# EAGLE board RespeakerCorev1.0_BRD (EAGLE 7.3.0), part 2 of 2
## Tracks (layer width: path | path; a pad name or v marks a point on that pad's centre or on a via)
!PWR_ON  (via drill 0.25 pad 0.51)
  Top 0.152: J6.P$14 J6.14 61.1,28.72 61.4,29.02 61.4,30.67 60.64,31.43 60.64,41.08 57.84,43.88 v57.46,43.88
  Bottom 0.152: v57.46,43.88 57.84,44.26 57.84,49.59 57.43,50.01 Q4.3 56.83,51.52 R4.1 D20.+ 54.65,52.08 Q3.1 54.53,51.09 C27.1
AGND  (via drill 0.25 pad 0.51)
  Top 0.203: U8.8 48.71,21.6 v48.95,21.84 | U8.7 48.9,21.2 v48.95,21.15 | U8.3 46.96,20.42 46.8,20.26 46.29,20.26 v46.16,20.38
  Top 0.406: 44.38,20.87 C68.1 44.41,21.38 v44.38,21.4 44.41,21.42 C69.1 | C29.1 48.93,23.58 48.95,23.56 | 48.95,23.56 48.95,23.58 | 48.95,23.69 48.95,23.58 | 48.95,23.58 R31.1 | 48.95,23.56 48.95,22.65 | C37.1 38.56,27.47 v38.41,27.62 | v45.78,25.21 45.78,24.6 C28.1 | R30.1 C28.1 | C28.1
  Top 0.508: MIC1.2 MIC1.3 | 48.99,21.88 R47.1 50.45,21.88 v50.48,21.91 | 48.99,21.88 v48.95,21.84 | 48.95,22.65 48.95,21.92 48.99,21.88
  Top 0.61: J2.4 39.09,1.63 v40.32,2.86 | J2.3 44.56,2.43 v43.75,3.24 | v38.41,27.62 38.41,28.05 MIC1.3 | MIC1.2 35.83,27.75 C18.1
  Top 1.016: J6.13 J6.P$13
  GND 1.016: J6.P$13 49.89,28.72 49.72,28.89
  Bottom 0.254: U5.28 37.65,38.92 v37.4,38.67
  Bottom 0.406: v45.27,46.42 45.29,46.4 R34.2 47.03,46.4 v47.05,46.42 48.07,45.4 v48.07,45.28 | C24.1 42.22,35.88 v42.35,35.75 | U4.1 v47.81,41.97 | v47.81,41.97 | C15.1 48.07,42.23 v47.81,41.97 | C15.1 v47.3,42.74 46.54,43.5 C14.1 | C15.1 v48.07,43.5 | v48.07,43.5 | C16.1 v48.07,43.5 | v48.07,43.5 | C16.1 v48.07,45.28 | v48.07,45.28 | C14.1 v46.16,44.51 | v46.16,44.51 | C14.1 | v44.64,44.51 C13.1 C14.1 | v44.64,44.51 | C14.1 | v44.64,44.51 v46.16,44.51 | v46.16,44.51 47.94,44.51 C16.1 | C54.2 42.73,40.96 v42.6,41.08 | C38.1 C39.1
  Bottom 0.508: C55.1 v42.6,41.08 | C54.2 v43.49,39.81
  Bottom 0.61: v40.83,33.08 40.8,33.11 C53.1 39.53,32.45 C52.2 38.92,31.46 C39.1 | C38.1 38.54,30.06 38.54,27.75 v38.41,27.62
  other vias: 35.87,38.67 34.35,38.67 34.35,40.2 35.87,40.2 37.4,40.2 37.4,37.15 35.87,37.15 34.35,37.15
  pour GND (isolate 0.254): 39.94,2.6 44.38,2.6 44.38,12.38 51.24,19.24 51.24,43.04 47.22,47.05 40.76,47.05 33.94,40.23 33.94,36.39 44.13,26.19 44.13,16.33 39.94,12.13
AVDD  (via drill 0.25 pad 0.51)
  Top 0.203: U8.1 46.21,21.6 v45.91,21.91
  Top 0.406: v45.91,21.91 C69.2 | v35.62,24.83 35.9,24.83 R58.1
  PWR 0.61: v49.59,43.62 v49.59,41.97 | v49.59,41.97 | 42.29,33.27 42.73,33.72 | 42.73,33.72 49.59,40.58 v49.59,41.97 | v41.46,34.1 41.84,33.72 | 41.84,33.72 42.29,33.27 | 41.84,32.83 35.62,26.61 v35.62,24.83 | 41.84,32.83 42.29,33.27 | 41.84,32.83 41.84,33.72 | 41.84,33.72 42.73,33.72
  Bottom 0.254: U5.32 39.68,36.92
  Bottom 0.406: 40.7,35.9 40.7,35.12 TP4.T | 40.7,35.9 39.68,36.92 | C24.2 40.7,35.9 | v35.62,24.83 41.72,24.83 44.38,22.16 45.65,22.16 v45.91,21.91
  Bottom 0.61: C16.2 v49.59,43.62 C15.2 | C15.2 | U4.2 v49.59,41.97 C15.2 | C15.2 | TP4.T v41.46,34.1
GND  (via drill 0.25 pad 0.51)
  Top 0.152: LC4.1 26.56,65.68 arc-90 26.6,65.72 26.48,65.72 v28.19,66.48 | LC4.2 v27.11,62.8
  Top 0.254: C65.1 27.21,27.77 26.35,28.64 20,28.64 18.98,27.62 18.98,26.23 19.24,25.97 C64.1 18.62,25.82 v18.6,25.84 | v24.63,10.86 24.63,11.3 22.79,13.14 22.49,13.14 | C41.1 22.25,12.92 v22.48,13.14
  Top 0.305: D7.2 27.11,8.32 v26.73,8.7 | D6.2 28.51,8.32 v28.89,8.7 | U7.5 23.69,20.52 v24.19,21.02 | U7.43 22.19,20.29 v22.92,21.02 | U7.15 25.73,21.29 v25.46,21.02 | U7.23 26.69,26 v26.98,26.29 | U7.33 21.69,25.8 21.52,25.97 v21.27,25.97 | U7.35 22.19,24.29 v22.92,23.56 | 30.98,27.05 v30.92,26.99 30.83,26.9 Q1.2 | C67.1 17.9,20.7 v17.84,20.76 | v17.84,20.76 17.84,20.19 17.71,20.07 | v17.84,20.76 17.84,21.4
  Top 0.406: C17.1 33.12,10.69 v33.08,10.73
  Top 0.5: 14.66,61.47 15.03,61.73 arc-20 15.2,61.81 v15.55,61.91
  Top 0.508: C62.1 23.96,16.17 24.77,15.35 | C65.1 27.21,26.52 v26.98,26.29 | C2.1 30.94,27.01 v30.92,26.99 | U6.31 50.76,32.03 | C67.1 18.37,21.12 v18.22,21.27 | C74.2 25.13,15.35 25.71,15.94 v25.97,15.94 | C45.1 25.31,56.3 v25.59,56.58
  Top 0.61: C74.2 24.77,15.35
  Top 0.813: v47.56,2.35 45.65,2.35 v45.65,3.75 | v36.51,1.71 38.54,1.71 v38.54,2.86
  Bottom 0.254: U5.20 35.62,42.35 v35.49,42.48 | U5.24 37.62,41.69 v37.65,41.72 | U5.9 33.11,36.92 32.83,36.64 v32.83,35.62
  Bottom 0.305: U2.3 18.22,14.29 U2.9 | U2.1 19.22,14.3 18.98,14.54 18.86,14.54 U2.9 | U2.6 18.22,14.79 U2.9 | U1.5 U1.PAD | U1.PAD | U2.9 | Q4.2 57.53,51.21 v57.68,51.36
  Bottom 0.406: C49.2 v41.21,46.16 | C33.1 v39.18,46.55 | 18.86,14.54 19.74,14.54 19.87,14.41 | U2.9 17.2,14.54 | v44.32,59.69 44.51,59.5 44.51,57.85 | C48.1 v30.67,10.48
  Bottom 0.508: C51.1 v42.6,42.1 | R6.1 28.23,14.57 C10.1 28,15.18 v27.24,15.94 | C50.1 v36,45.66 | C56.2 42.68,19.65 C57.2 | C5.1 23.17,7.43 v23.3,7.3 | J7.6 43.44,17.03 v43.49,17.08 | R56.1 37.5,17.74 v37.91,17.34
  Bottom 0.61: 27.62,10.73 27.49,10.86 U1.PAD 23.68,10.86 | J7.G1 48.04,14.52
  other vias: 33.84,47.43 46.92,45.4 45.27,45.4 24.95,34.99 28.38,37.66 24.89,46.99 29.71,58.42 29.97,59.05 31.49,62.61 41.4,59.56 46.48,59.69 48.64,55.5 51.94,52.45 51.81,51.05 51.94,49.02 51.81,47.5 60.07,47.5 52.13,32.51 25.71,10.86 20.13,31.69 6.66,36.26 8.31,28.77 9.01,43.31 18.47,14.54 16.44,16.19 13.65,16.32 13.65,15.3 17.14,14.54 19.81,14.41 15.62,10.22 21.08,13.14 26.54,10.92 32.06,14.8 31.43,5.52 24.7,5.4 58.86,17.08 64.58,17.59 58.23,22.8 58.23,24.07 5.52,17.59 6.28,16.19 8.7,21.4 50.16,16 20.76,8.32 44.57,49.4 63.69,16.19 26.86,1.33 23.3,35.75 26.73,48.45 29.14,10.48 49.65,57.98 60.45,54.04 52.83,15.94 57.91,10.86 19.81,5.78 14.73,8.32 12.19,10.86 7.68,20.38 24.25,43.88 27.94,49.47 52.83,18.48 23.68,4.38 25.08,49.47 24.06,37.66 43.24,48.2 46.67,48.2 26.6,15.94 30.73,19.81 31.43,21.78 24.19,22.29 25.46,22.29 22.92,22.29 25.46,23.56 24.19,23.56 47.75,62.61 43.43,62.48 43.94,63.25 46.99,63.25 17.84,19.62 18.92,9.21 20.25,25.84 57.21,45.15 54.03,54.04 8.38,40.7 6.98,40.07 13.33,45.15 54.61,7.05 29.9,8.95 23.81,10.6 23.3,48.32 49.59,61.66 55.88,57.34 54.61,57.21 62.73,50.23 38.79,55.31 45.97,55.94 6.98,25.46 8.25,27.37 9.01,44.64 11.49,20.13 11.49,24.19 54.03,10.22 18.98,56.83 19.49,55.69 21.01,55.31 22.28,55.31 23.55,55.31 23.55,52.77 22.28,52.77 21.01,52.77 19.74,53.4 18.35,54.17 10.54,49.72 63.43,37.02 64.07,32.07 63.75,31.05 21.65,9.59 21.78,10.99 15.43,16.13 25.78,60.58 24.25,60.07 17.01,59.75 18.16,52.9 20.19,52.39 21.01,51.5 22.28,51.5 23.55,51.5 21.9,59.37 29.52,61.79 52.32,13.78 19.11,63.18 11.74,50.36 14.03,50.36 8.31,23.49 4.5,21.59 5.77,23.56 21.65,43.88 62.35,43.24 63.75,29.27 62.67,26.1 62.29,23.56 61.65,19.11 61.02,13.4 21.71,12.64 21.08,12.38 20.19,13.78 42.6,56.96 17.46,55.31 27.62,61.15 16.95,56.58 18.98,58.48 15.93,57.21 18.98,59.75 15.17,57.85 15.17,58.99 25.21,62.17 23.17,61.4 19.74,61.02 23.43,28.57 27.72,26.72 21.27,60.64 29.02,63.56 59.97,51.74 62.63,52.88 57.93,57.96 28.89,12.83 17.33,62.55 29.97,67.12 32,67.88 28.82,65.09 30.6,65.72 32.51,66.36 30.98,64.2 15.87,59.75 17.14,61.15 15.87,61.02 56.22,49.64 55.9,47.17 57.04,47.17 28.44,57.53 64.54,49.9 36.57,62.99 40.38,64.64 41.91,65.79 38.98,65.79 40.13,67.18 7.3,52.9 4.5,48.07 34.1,32.58 30.92,36.13 31.43,14.8 43.49,19.49 30.92,23.81 30.16,23.81 28.38,38.29 49.4,10.99 20.13,32.45 18.41,32.64 29.52,6.54 30.29,6.54 31.05,6.54 29.9,5.91 30.67,5.91 50.8,53.34 49.65,52.45 50.8,51.56 51.05,49.91 51.05,48.26 49.65,47.37 50.8,46.61 49.84,49.4 49.84,51.05 48.64,52.83 49.27,53.72 47.87,53.72 18.16,51.88 18.79,53.4 36,30.42 36,29.91 48.13,16.26 47.87,13.59 49.14,14.99 48,11.43 48.51,10.67 48.51,9.65 48.26,7.75 46.1,6.6 43.68,6.6 42.03,4.95 37.33,9.4 40,6.48 44.45,11.3 43.18,9.65 32.7,42.1 43.11,36.26 43.11,35.62 26.86,36.26 24.95,37.66 34.6,15.18 33.33,13.91 33.84,23.18 33.84,24.7 33.71,26.73 34.35,28.64 34.86,29.15 34.86,31.69 39.43,28.64
  pour Top (isolate 0.254, rank 6): -2.23,-3.62 71.81,-3.62 71.81,70.42 -2.23,70.42
  pour GND (isolate 0.254, rank 5): -2.23,48.96 -2.23,-4.38 -0.58,-4.38 -0.58,-3.62 71.81,-3.62 71.81,70.42 8.57,70.42 -1.49,70.39 -2.22,70.4 -2.22,62.44 -2.23,50.29 -2.23,49.43
  pour Bottom (isolate 0.254, rank 5): -2.23,70.42 -2.23,-5.65 -0.58,-5.65 -0.58,-3.62 71.81,-3.62 71.81,70.42
  pour Top (isolate 0.254, rank 3, no thermals): 22.92,5.52 32.44,5.52 32.44,-1.84 22.92,-1.84
  pour Top (no thermals): 28.51,64.07 27.62,66.48 32.7,68.39 33.59,66.1
  pour Top (no thermals): 27.75,65.85 28.38,64.07 20.44,61.15 20.13,61.91 19.87,61.85 20.51,60.26 29.46,63.56 28.51,66.23 27.75,65.98
  pour Top (isolate 0.254, rank 4, no thermals): 15.17,60.01 14.16,61.79 19.74,63.69 21.01,60.52
GPIO12/UART_TXD0  (via drill 0.25 pad 0.51)
  Top 0.152: 30.03,30.67 30.03,30.57 U6.19 | J6.4 J6.P$4
  Top 0.203: 30.03,30.67 v30.03,31.31
  PWR 0.152: v60.89,29.27 60.89,36.26 58.43,38.72 J6.P$4
  Bottom 0.152: v30.03,31.31 34.86,26.48 42.35,26.48 45.14,23.69 50.61,23.69 52.43,25.51 58.28,25.51 60.89,28.13 v60.89,29.27
  Bottom 0.203: v30.03,31.31 29.4,31.94 TP16.T
GPIO13/UART_RXD0  (via drill 0.25 pad 0.51)
  Top 0.152: U6.20 31.58,30.64 30.92,31.31 v30.79,31.31 | J6.3 J6.P$3
  PWR 0.152: v60.38,29.91 60.38,36.26 58.86,37.78 56.51,37.78 J6.P$3
  Bottom 0.152: v60.38,29.91 60.38,28.13 58.1,25.84 52.26,25.84 50.48,24.07 45.27,24.07 42.48,26.86 34.98,26.86 30.79,31.05 v30.79,31.31 31.43,31.94 TP17.T
GPIO_0/I2S_ADC  (via drill 0.25 pad 0.51)
  Top 0.152: U6.7 18.98,42.23 17.84,41.08 17.84,40.58 16.95,39.69 13.9,39.69 13.39,39.18 13.39,37.72 J5.P$5 J5.5
  Top 0.203: U6.7 v20.38,42.23 | v20.38,42.23
  PWR 0.203: v20.38,42.23 22.12,40.48 v32.57,40.48
  Bottom 0.203: U5.16 32.64,40.42 v32.57,40.48
GPIO_1/I2S_DAC  (via drill 0.25 pad 0.51)
  Top 0.152: U6.8 18.93,40.53 17.12,38.72 J5.4 J5.P$4
  Top 0.203: U6.8 20.33,40.53 v20.38,40.58
  PWR 0.203: v32.57,39.43 21.52,39.43 v20.38,40.58
  Bottom 0.203: U5.14 v32.58,39.42 v32.57,39.43
GPIO_2/I2S_LRCLK  (via drill 0.25 pad 0.51)
  Top 0.152: U6.9 18.88,38.83 16.78,36.72 J5.6 J5.P$6
  Top 0.203: U6.9 20.28,38.83 v20.38,38.93
  PWR 0.203: v20.38,38.93 v20.38,38.92 v32.07,38.92
  Bottom 0.203: v32.07,38.92 U5.13
GPIO_3/I2S_BCLK  (via drill 0.25 pad 0.51)
  Top 0.152: v20.38,37.91 19.6,37.13 U6.10 18.84,37.13 16.43,34.72 J5.8 J5.P$8
  PWR 0.203: v27.5,38.36 20.83,38.36 v20.38,37.91
  Bottom 0.203: R40.2 29.02,39.94 27.5,38.42 v27.5,38.36
GPIO_4/I2C_SCL  (via drill 0.25 pad 0.51)
  Top 0.152: U6.11 19.04,35.43 16.33,32.72 J5.10 J5.P$10
  Top 0.203: U6.11 20.06,35.43 v20.13,35.5
  Bottom 0.203: U5.17 34.12,41.44 33.97,41.59 32.19,41.59 31.56,42.23 R39.1 30.77,42.51 30.41,42.86 27.68,42.86 21.34,36.52 20.39,36.52 20.13,36.26 v20.13,35.5
GPIO_5/I2C_SDA  (via drill 0.25 pad 0.51)
  Top 0.152: U6.12 18.23,33.73 17.84,33.34 17.84,32.07 16.49,30.72 J5.12 J5.P$12
  Top 0.203: U6.12 20.01,33.73 20.76,34.48 v20.76,37.15
  Bottom 0.203: U5.18 34.62,41.45 34.1,41.97 33.59,41.97 33.21,42.35 R38.1 arc90 33.1,43.24 27.24,43.24 21.14,37.15 v20.76,37.15
GPIO_19/PWM_CH1  (via drill 0.25 pad 0.51)
  Top 0.152: U6.34 49.1,37.13 v48.32,37.91
  Bottom 0.152: BUTTON1.1 39.24,60.96 40.32,59.88 40.32,58.4 43.92,54.8 56.57,54.8 57.09,54.29 R33.1 58.28,53.4 TP15.T 59.58,53.45 61.54,51.49 K2.2 61.54,49.81 K2.1 63.25,48.01 59.11,43.88 59.11,40.7 58.1,39.69 54.03,39.69 52.26,37.91 v48.32,37.91
GPIO_40  (via drill 0.25 pad 0.51)
  Top 0.152: U6.57 26.48,53.78 27.62,52.64 v27.62,51.75
  Bottom 0.152: D21.- 52.38,47.69 48.32,51.75 v27.62,51.75
GPIO_41
  Top 0.152: U6.2 18.85,50.73 17.46,49.34 16.67,48.55 R48.1
GPIO_42  (via drill 0.25 pad 0.51)
  Top 0.152: U6.58 24.78,54.31 24.82,54.35 24.82,54.42 v25.46,55.05
  Bottom 0.152: 53.27,52.3 D20.- 53.23,52.81 51.75,54.29 43.75,54.29 40.38,57.66 R11.1 39.29,58.91 TP6.T 37.17,58.96 35.17,60.96 BUTTON1.2 34.92,60.96 29.02,55.05 v25.46,55.05
GPIO_45/UART_TXD1
  Top 0.152: J5.P$1 17.3,45.63 U6.5 | J5.P$1 | J5.1 J5.P$1
GPIO_46/UART_RXD1
  Top 0.152: U6.6 16.19,43.93 13.39,41.13 13.39,39.69 12.43,38.72 J5.P$3 J5.3
HP_L  (via drill 0.25 pad 0.51)
  Top 0.203: U8.4 47.36,20.06 v47.05,19.75
  Top 0.61: J6.7 J6.P$7 | L4.1 45.85,17.53 D15.1 45.88,18.51 45.88,18.61 45.91,18.61 v47.05,19.75
  PWR 0.61: v47.05,19.75 47.05,23.94 49.34,26.23 v49.34,27.37
  Bottom 0.61: v49.34,27.37 49.34,29.15 50.35,30.16 50.35,33.59 51.3,34.54 51.37,34.61 51.48,34.72 J6.P$7
HP_R  (via drill 0.25 pad 0.51)
  Top 0.203: U8.5 47.76,20.06 v48.07,19.75
  Top 0.406: J6.8 J6.P$8
  Top 0.61: L2.1 47.11,17.27 47.11,18.35 D16.1 47.23,18.79 48.07,19.62 v48.07,19.75
  PWR 0.61: v48.07,19.75 48.07,23.69 50.22,25.84 v50.22,27.37
  Bottom 0.406: J6.P$8 56.57,33.72 54.8,33.72
  Bottom 0.61: v50.22,27.37 50.22,28.77 51.24,29.78 51.24,32.96 52,33.72 54.8,33.72
HP_SEL  (via drill 0.25 pad 0.51)
  Top 0.152: U8.6 49.4,20.6 R47.2 50.76,20.92 v52.13,22.29 | J6.2 J6.P$2 | R48.2 15.68,48.2 v14.66,47.18
  PWR 0.152: v52.13,22.29 52.13,24.32 52.76,24.96 60.64,24.96 61.4,25.72 61.4,36.89 J6.P$2
  Bottom 0.152: v14.66,47.18 15.05,47.56 24.44,47.56 28,51.12 47.3,51.12 57.57,40.85 J6.P$2
LIN1
  Bottom 0.305: U5.4 36.12,35.75 36.13,35.75 36.13,35.24
  Bottom 0.406: C36.2 35.87,34.99 36.13,35.24
MCLK_OUT  (via drill 0.25 pad 0.51)
  Top 0.152: v17.2,40.7 17.19,40.72 J5.2 J5.P$2
  PWR 0.203: v31.94,39.94 21.9,39.94 20.51,41.34 17.84,41.34 v17.2,40.7
  Bottom 0.203: v31.94,39.94 33.4,39.94 U5.15
MIC_VDD
  Top 0.406: R58.2 37.92,24.57 39.43,26.08 C37.2
  Top 0.61: C18.2 36.08,26.23 MIC1.1 37.12,25.18 R58.2 R57.2
MICBIAS  (via drill 0.25 pad 0.51)
  Top 0.61: R57.1 35.49,23.56 v34.73,24.32
  PWR 0.61: v39.74,34.71 39.74,32.38 34.73,27.37 v34.73,24.32
  Bottom 0.254: U5.1 37.62,35.52 | TP13.T
  Bottom 0.406: C53.2 39.68,34.08 | 39.68,34.08 39.02,34.08 C52.1 38.92,34.23 37.62,35.52 | v39.74,34.71 39.74,34.13 39.68,34.08 | v39.74,34.71 39.74,34.55 40.19,34.1 | v39.74,34.71 39.74,34.66 39.18,34.1 | TP13.T 39.18,35.27 v39.74,34.71
MT_GPIO0  (via drill 0.25 pad 0.51)
  Top 0.152: U6.18 28.18,31.5 v28.13,31.56 | R2.2 v28.89,28.51
  PWR 0.152: v28.89,28.51 28.89,30.8 v28.13,31.56
MT_GPIO_14/SPIS_CS  (via drill 0.25 pad 0.51)
  Top 0.152: U6.39 51.85,45.63 v51.88,45.66 | U7.8 25.19,18.09 v25.36,17.92
  PWR 0.152: v25.36,17.92 26.17,18.73 30.35,18.73 50.22,38.61 50.22,44.01 v51.88,45.66
MT_GPIO_18/PWM_CH0
  Top 0.152: U6.35 51.34,38.83 53.45,36.72 J6.5 J6.P$5
MT_GPIO_39  (via drill 0.25 pad 0.51)
  Top 0.152: U7.1 21.69,18.65 v21.27,18.22 | U6.4 18.37,47.33 v17.97,46.93
  Bottom 0.152: v21.27,18.22 19.11,18.22 18.73,18.61 18.73,21.53 22.16,24.96 22.16,28.38 18.98,31.56 18.98,45.91 v17.97,46.93
MT_SPIS_CLK  (via drill 0.25 pad 0.51)
  Top 0.152: v26.09,17.72 26.09,17.97 25.69,18.38 U7.9 | U6.38 51.16,43.93 v51.75,44.51
  PWR 0.152: v26.09,17.72 26.73,18.35 30.41,18.35 50.61,38.54 50.61,43.37 v51.75,44.51
  Bottom 0.152: TP5.T v26.09,17.72
MT_SPIS_MISO  (via drill 0.25 pad 0.51)
  Top 0.152: U6.37 50.73,42.23 v51.49,41.47 | U7.11 26.69,18.65 v27.49,17.84
  PWR 0.152: v51.49,41.47 50.99,40.96 50.99,38.48 30.48,17.97 27.62,17.97 v27.49,17.84
  Bottom 0.152: v27.49,17.84 30.29,17.84 TP8.T
MT_SPIS_MOSI  (via drill 0.25 pad 0.51)
  Top 0.152: U7.10 26.19,18.35 27.36,17.18 v27.36,16.95 | U6.36 51.7,40.53 v51.88,40.7
  PWR 0.152: v27.36,16.95 28,17.59 30.54,17.59 51.49,38.54 51.49,40.32 v51.88,40.7
  Bottom 0.152: TP7.T v27.36,16.95
MT_UART_RXD  (via drill 0.25 pad 0.51)
  Top 0.152: U7.21 28.22,24.29 29.4,25.46 31.81,25.46 33.21,24.07 33.21,19.11 v34.22,18.1 | 50.49,33.73 U6.32 52.12,33.73 52.64,33.21 v52.64,31.94
  PWR 0.152: v52.64,31.94 47.94,31.94 34.22,18.22 v34.22,18.1
  Bottom 0.152: TP25.T 35.37,19.62 34.22,18.48 v34.22,18.1
MT_UART_TXD  (via drill 0.25 pad 0.51)
  Top 0.152: U7.20 28.23,23.79 29.52,25.08 31.68,25.08 32.83,23.94 32.83,18.48 v33.84,17.46 | U6.33 51.68,35.43 v52.13,35.88
  PWR 0.152: v52.13,35.88 53.27,34.73 53.27,31.81 52.89,31.43 47.94,31.43 34.73,18.22 34.73,17.84 34.35,17.46 v33.84,17.46
  Bottom 0.152: TP24.T 34.35,17.46 v33.84,17.46
N$1
  Bottom 0.152: R46.1 53.42,48.85 54.58,50.01 Q3.3
N$2
  Top 0.152: 21.4,53.94 21.37,53.94 21.27,54.04 U6.60 | U6.60
  Top 0.5: U6.60 21.15,54.03 arc-90 17.98,57.2 LC3.2 16.9,57.91 LC2.2
N$3
  Bottom 0.152: R12.1 53.25,58.64 D11.1
N$4
  Top 0.203: U8.2 45.68,21.2 C68.2
N$5
  Bottom 0.203: U5.11 30.02,37.92 C75.2 R49.1
N$6  (via drill 0.25 pad 0.51)
  Top 0.406: MIC1.4 37.65,26.35 v37.65,27.37
  Bottom 0.406: L8.1 35.87,31.56 37.27,30.16 C38.2 37.68,27.39 v37.65,27.37
N$7
  Bottom 0.152: D12.1 50.72,56.92 R17.1
N$8
  Top 0.152: R10.1 28.38,10.48 28,10.86 28,12 26.98,13.02 24.06,13.02 22.92,14.16 22.92,17.46 23.19,17.73 U7.4
N$9  (via drill 0.25 pad 0.51)
  Top 0.152: R32.1 43.49,26.35 36.64,19.49 36.64,15.43 36.13,14.92 v36.13,14.03
  Bottom 0.152: J7.5 42.34,14.41 41.84,13.91 36.25,13.91 v36.13,14.03
N$10
  Top 0.152: R9.1 27.24,10.48 27.62,10.86 27.62,11.87 26.86,12.64 23.94,12.64 22.54,14.03 22.54,17.59 22.69,17.74 U7.3
N$11
  Top 0.152: D9.1 18.05,11.45 17.33,10.73 13.52,10.73 11.68,12.57 11.62,12.64 11.18,13.07 D10.3
N$12
  Bottom 0.254: R6.2 26.09,12.76 25.71,12.38 U1.2 | U1.2
N$13
  Top 0.152: D19.1 46.59,60.34 47.81,59.12 D1.3 | 47.68,59.12 D1.3 | D1.3
N$14
  Bottom 0.254: U5.22 36.62,41.96 37.4,42.74 L6.1
N$15  (via drill 0.25 pad 0.51)
  Top 0.203: J1.2 27.51,5.8 27.62,5.91 27.62,7.3 | 27.62,7.3 27.56,7.36 D7.1 v27.11,6.92 | 27.62,7.3 27.62,9.1 R9.2
  Bottom 0.152: v27.11,6.92 27.11,7.3 TP19.T
N$16  (via drill 0.25 pad 0.51)
  Top 0.203: J1.3 28.16,5.75 28,5.91 28,7.43 | 28,7.43 28,9.1 R10.2 | 28,7.43 28.07,7.36 D6.1 v28.51,6.92
  Bottom 0.152: TP20.T v28.51,6.92
N$17
  cutout GND (isolate 0.254): 56.32,60.22 52.45,62.93 51.27,61.23 55.14,58.52
  cutout PWR (isolate 0.254): 52.84,62.66 52.46,62.92 51.27,61.23 55.14,58.52 56.32,60.22
N$18
  Top 0.152: D10.1 11.12,23.05 6.61,27.56 D13.3
N$19  (via drill 0.25 pad 0.51)
  Top 0.152: D9.3 22.16,7.94 v21.9,7.68 | D8.1 33.68,5.49 v33.71,5.52
  PWR 0.152: v21.9,7.68 22.41,8.19 31.05,8.19 v33.71,5.52
N$20
  Bottom 0.152: R20.2 4.63,35.12 J13.1
N$21
  Bottom 0.152: C19.2 R3.1 | R3.1 54.44,48.81 54.42,48.83 R46.2 54.39,48.13 D21.+ | Q4.1 55.94,50.72 55.92,50.72 55.69,50.48 55.69,49.06 R3.1
N$22
  Bottom 0.152: R18.2 7.68,38.16 J14.1
N$23
  Top 0.152: D14.3 7.81,44.74 7.81,36 8.36,35.45 D13.1
N$24
  Bottom 0.406: C36.1 L8.2 37.4,31.46 C39.2
N$25  (via drill 0.25 pad 0.51)
  Top 0.152: v21.4,58.48 20.8,58.48 D18.3 | D14.1 13.6,48.4 v13.78,48.58
  Bottom 0.152: v21.4,58.48 24.19,55.69 24.19,50.74 22.03,48.58 v13.78,48.58
N$26
  Bottom 0.203: R40.1 C20.2 30.64,38.29 32.19,38.29 32.32,38.42 U5.12
N$27  (via drill 0.25 pad 0.51)
  Top 0.152: U6.14 21.38,30.66 21.9,31.18 v21.9,31.43
  Bottom 0.152: v21.9,31.43 21.9,32.7 TP9.1
N$28
  Top 0.152: Q1.1 29,26.9 R2.1
N$29
  Bottom 0.025: L1.1 19.25,11.11
  pour Bottom (no thermals): 18.63,14.16 18.77,14.16 18.86,14.07 18.86,13.27 19.49,12.64 19.49,10.57 19.4,10.48 18.63,10.48 18.54,10.57 18.54,14.07
N$30
  Top 0.152: D19.3 31.95,60.64 29.52,60.64 27.87,58.99 24.85,58.99 D18.1
N$31
  Bottom 0.152: R41.2 65.34,35.12 J8.1
N$32  (via drill 0.25 pad 0.51)
  Top 0.305: v16.06,11.87 16.95,11.87 v17.97,12.89
  Bottom 0.203: U2.4 17.71,13.7
  Bottom 0.305: R5.1 14.43,10.88 15.4,11.85 R7.2 16.04,11.85 v16.06,11.87 | 17.71,13.7 17.71,13.14 v17.97,12.89
N$33
  Bottom 0.152: R21.2 5.52,33.21 J12.1
N$34
  Bottom 0.152: R23.2 9.23,31.08 4.5,26.35 J11.1
N$35
  Bottom 0.152: R43.2 62.16,37.15 65.46,40.45 J3.1
N$36
  Bottom 0.152: R36.2 64.7,32.96 J9.1
N$37
  Bottom 0.152: R19.2 62.14,29.42 J10.1
N$38
  Bottom 0.254: U5.19 35.12,41.96 34.6,42.48 L7.1
N$39  (via drill 0.25 pad 0.51)
  PWR 0.406: v36.51,47.82 v44.64,55.94
  Bottom 0.406: L6.2 37.4,46.52 C33.2 C31.1 36.48,47.79 v36.51,47.82 | J4.1 46.06,63.9 C35.2 45.78,62.27 45.78,57.09 v44.64,55.94
N$40
  Top 0.305: U7.6 24.19,18.22 23.68,17.72 C62.2
N$41  (via drill 0.25 pad 0.51)
  Top 0.305: C67.2 19.43,20.79 19.91,20.79 v19.93,20.76 19.96,20.79 U7.42
  Bottom 0.305: v19.93,20.76 20.63,20.76 TP27.T
N$42
  Top 0.152: D1.1 55.23,56.01 58.76,52.48 D2.3
N$43  (via drill 0.25 pad 0.51)
  Top 0.305: U7.44 19.91,19.79 19.87,19.75 | U7.24 26.19,26.57 v26.22,26.61
  Top 0.508: FB2.2 v19.24,18.99 19.24,19.52 C66.2 19.47,19.75 19.87,19.75 | C65.2 26.25,26.63 v26.22,26.61
  Bottom 0.508: v19.24,18.99 19.24,21.29 23.92,25.97 25.59,25.97 v26.22,26.61
N$44
  Top 0.152: D3.3 63.34,35.53 63.94,36.13 63.94,38.29 58.83,43.4 D2.1
N$45
  Top 0.152: D4.3 60.32,20.83 61.78,22.29 61.78,31.95 D3.1
N$46
  Top 0.152: D4.1 57.21,12.13 53.78,8.7 50.99,8.7 50.76,8.93 D5.3
N$47  (via drill 0.25 pad 0.51)
  PWR 0.406: v35.62,47.82 v43.87,56.07
  Bottom 0.406: L7.2 34.6,46.52 C32.2 35.49,46.55 | 35.49,46.55 C31.2 | J4.2 44.99,65.09 C34.2 45.14,62.4 45.14,57.34 v43.87,56.07 | 35.49,46.55 35.56,46.61 35.56,47.75 v35.62,47.82
N$49
  Top 0.305: U7.17 28.63,22.29 29.33,22.98 X3.1
N$50
  Top 0.305: U7.16 28.37,21.79 29.58,20.58 X3.3
N$51
  Top 0.5: ANT1.ANT 19.55,62.42 arc60 17.98,60.52 LC3.1 16.93,58.88 LC1.2
N$52  (via drill 0.25 pad 0.51)
  Top 0.152: U6.15 23.08,30.76 22.67,31.18 v22.67,31.43
  Bottom 0.152: v22.67,31.43 22.67,32.7 TP10.1
N$53  (via drill 0.25 pad 0.51)
  Top 0.152: U6.16 24.78,30.76 25.21,31.18 v25.21,31.43
  Bottom 0.152: v25.21,31.43 25.21,32.7 TP11.1
N$54  (via drill 0.25 pad 0.51)
  Top 0.152: U6.17 26.48,30.66 25.97,31.18 v25.97,31.43
  Bottom 0.152: v25.97,31.43 25.97,32.7 TP22.1
N$55
  cutout PWR: 15.17,62.11 14.16,64.13 31.25,70.93 32.25,68.27 32.7,66.99 33.46,65.21 34.35,62.67 18.03,56.52
  cutout GND: 15.17,62.11 14.16,64.13 31.25,70.93 32.25,68.27 27.36,66.48 28.25,64.2 20.63,61.4 19.81,63.75
N$57  (via drill 0.25 pad 0.51)
  Top 0.203: U8.12 46.96,22.63 46.8,22.8
  Top 0.61: 46.8,22.8 46.77,22.82 R30.2 C28.2 v46.77,26.05
  Bottom 0.61: v46.77,26.05 46.77,29.93 46.1,30.61 46.03,30.67 45.78,30.92 C26.2
N$58
  Bottom 0.254: U5.29 39.17,38.42 39.18,38.42
  Bottom 0.61: C25.1 47.94,34.23 47.3,34.86 47.3,36.77 45.65,38.42 39.18,38.42 39.05,38.42
N$59  (via drill 0.25 pad 0.51)
  Top 0.152: D8.3 35.24,8.06 v35.24,8.83
  Bottom 0.152: U3.4 32.3,13.54 35.24,10.6 v35.24,8.83
N$60
  Bottom 0.254: U5.31 38.94,37.42 39.11,37.59
  Bottom 0.61: C26.1 45.78,34.23 46.41,34.86 46.41,36.39 45.21,37.59 39.11,37.59
N$61  (via drill 0.25 pad 0.51)
  Top 0.203: U8.10 47.76,22.87 47.81,22.92
  Top 0.61: 47.81,22.92 47.96,23.07 R31.2 C29.2 v47.96,26.08
  Bottom 0.61: v47.96,26.08 47.96,30.57 C25.2
N$63
  Top 0.61: 45.5,9.49 45.53,9.46 45.53,9.5 J2.2 45.5,9.58 C72.2 45.5,15.66 L4.2
N$64
  Top 0.61: L2.2 47.05,15.05 | 47.05,15.05 47.05,11.11 47.67,10.49 47.67,8.56 46.67,7.56 42.73,7.56 40.4,5.23 J2.5 38.56,6.55 C71.2 | 47.05,15.05
PB4/A8/D8  (via drill 0.25 pad 0.51)
  Top 0.152: U7.28 24.19,26.35 22.54,28 v21.65,28
  Bottom 0.152: R13.1 R23.1 11.59,29.78 17.71,29.78 18.73,28.77 18.73,27.11 19.49,26.35 20.89,26.35 21.65,27.11 v21.65,28
PB5/A9/D9  (via drill 0.25 pad 0.51)
  Top 0.152: U7.29 23.69,26.34 22.67,27.37 v21.14,27.37
  Bottom 0.152: R14.1 R21.1 11.59,31.81 16.32,31.81 19.11,29.02 19.11,27.24 19.62,26.73 20.51,26.73 v21.14,27.37
PB6/A10/D10  (via drill 0.25 pad 0.51)
  Top 0.152: U7.30 23.19,26.21 22.6,26.8 20.82,26.8 20.38,27.24 v20.38,28
  Bottom 0.152: R18.1 R16.1 11.72,35.62 15.05,35.62 15.93,34.73 15.93,33.46 20.38,29.02 v20.38,28
PB7/D11  (via drill 0.25 pad 0.51)
  Top 0.152: U7.12 27.83,19.79 28,19.62 28,18.73 v29.65,17.08
  Bottom 0.152: v29.65,17.08 30.02,16.72 U3.1
PC7/D13  (via drill 0.25 pad 0.51)
  Top 0.152: U7.32 22.19,26.19 21.9,26.48 20.63,26.48 v19.74,27.37
  Bottom 0.152: R15.1 R20.1 11.59,33.72 15.05,33.72 19.74,29.02 v19.74,27.37
PD0/SCL/D3  (via drill 0.25 pad 0.51)
  Top 0.152: U7.18 28.25,22.79 29.78,24.32 31.43,24.32 32.06,23.69 32.06,17.97 33.71,16.32 v33.84,16.32 | J6.12 J6.P$12
  PWR 0.152: J6.P$12 56.73,31.56 55.05,31.56 54.16,30.67 48.07,30.67 35.62,18.22 35.62,17.53 34.41,16.32 v33.84,16.32
  Bottom 0.152: R8.1 R19.1 57.78,30.92 J6.P$12
PD1/SDA/D2  (via drill 0.25 pad 0.51)
  Top 0.152: U7.19 28.24,23.29 29.65,24.7 31.56,24.7 32.44,23.81 32.44,18.1 33.65,16.89 v34.22,16.89 | J6.10 J6.P$10
  PWR 0.152: J6.P$10 56.72,31.86 54.85,31.86 54.03,31.05 48,31.05 35.24,18.29 35.24,17.84 34.29,16.89 v34.22,16.89
  Bottom 0.152: R37.1 R41.1 61.02,35.12 58.99,33.08 58.97,33.08 58.61,32.72 J6.P$10
PD4/A6/D4  (via drill 0.25 pad 0.51)
  Top 0.152: U7.25 25.69,27.07 v25.46,27.31 | J6.11 J6.P$11
  PWR 0.152: v51.62,22.92 51.62,26.77 J6.P$11
  Bottom 0.152: R35.1 R36.1 61.15,32.96 59.88,31.69 56.54,31.69 J6.P$11 | v25.46,27.31 27.94,27.31 29.9,25.34 41.97,25.34 44.7,22.61 51.3,22.61 v51.62,22.92
PD6/A11/D12  (via drill 0.25 pad 0.51)
  Top 0.152: U7.26 25.19,26.65 v25.21,26.67 | J6.6 J6.P$6
  PWR 0.152: v60.38,25.46 59.88,25.97 59.88,34.42 J6.P$6
  Bottom 0.152: v25.21,26.67 24.95,26.92 24.95,27.5 25.33,27.88 27.87,27.88 30.03,25.72 42.1,25.72 44.89,22.92 50.86,22.92 52.76,24.83 59.75,24.83 v60.38,25.46
PD7/A7/D6  (via drill 0.25 pad 0.51)
  Top 0.152: U7.27 24.69,26.81 v24.19,27.31 | J6.9 J6.P$9
  PWR 0.152: v59.5,25.46 59.5,32.83 v58.61,33.72 56.57,33.72 J6.P$9
  Bottom 0.152: R42.1 R43.1 61.15,37.15 60.38,36.39 60.38,34.99 59.11,33.72 v58.61,33.72 | v59.5,25.46 59.19,25.16 52.59,25.16 50.73,23.3 45.02,23.3 42.22,26.1 30.16,26.1 28,28.26 25.08,28.26 24.19,27.37 v24.19,27.31
PF0/A5
  Top 0.152: U7.41 18.97,21.29 17.84,22.42 17.84,23.3 16.32,24.83 14.28,24.83 J5.P$15 J5.15
PF1/A4
  Top 0.152: U7.40 18.97,21.79 18.22,22.54 18.22,23.43 16.44,25.21 14.41,25.21 13.39,26.23 13.39,27.72 J5.P$13 J5.13
PF4/A3  (via drill 0.25 pad 0.51)
  Top 0.152: U7.39 18.98,22.29 18.6,22.67 18.6,23.56 16.44,25.72 v15.3,25.72 | J5.11 J5.P$11
  PWR 0.152: v15.3,25.72 13.9,25.72 13.39,26.23 13.39,29.72 J5.P$11
PF6/A1  (via drill 0.25 pad 0.51)
  Top 0.152: U7.37 19.38,23.29 v19.36,23.3 | J5.9 J5.P$9
  PWR 0.152: v19.36,23.3 19.11,23.3 15.55,26.86 15.55,31.18 15.05,31.69 13.43,31.69 J5.P$9
PF7/A0  (via drill 0.25 pad 0.51)
  Top 0.152: U7.36 18.88,23.79 17.71,24.96 v17.71,25.46 | J5.7 J5.P$7
  PWR 0.152: v17.71,25.46 17.46,25.46 15.93,26.99 15.93,32.45 14.66,33.72 13.39,33.72 J5.P$7
PORST_N  (via drill 0.25 pad 0.51)
  Top 0.254: C61.2 40.45,57.75 R53.1 R55.1 40.47,56.04 v40.57,55.94 40.08,55.46 U6.49
  Bottom 0.254: TP26.T 40.06,55.44 v40.57,55.94
PW_FAULT
  Bottom 0.152: U1.3 26.4,11.87
  Bottom 0.305: 26.4,11.87 TP21.T
REF_CLKO  (via drill 0.25 pad 0.51)
  Top 0.152: U6.46 45.18,53.06 v45.14,53.02
  PWR 0.203: v27.11,41.08 33.21,41.08 35.11,42.99 40.83,42.99 45.14,47.31 v45.14,53.02
  Bottom 0.203: R49.2 27.75,36.89 26.86,37.78 26.86,40.83 v27.11,41.08
RST_A  (via drill 0.25 pad 0.51)
  Top 0.152: R1.1 32.4,27.94 31.47,27.94 C2.2 30.77,27.98 v30.67,27.88 30.45,28.1 Q1.3 | U7.13 28.22,20.29 28.51,20 v28.51,19.75
  PWR 0.152: v28.51,19.75 28.51,25.72 v30.67,27.88
  Bottom 0.203: TP23.T 28.51,18.86 v28.51,19.75
SD_CD  (via drill 0.25 pad 0.51)
  Top 0.152: U6.24 38.38,30.57 38.79,30.16 38.79,29.78 39.3,29.27 40.21,29.27 40.95,28.53 40.95,25.34 35.49,19.88 35.49,16.07 v35.24,15.81
  Bottom 0.152: Q2.3 36.42,17.96 R56.2 36.53,17.11 v35.24,15.81
SD_CLK
  Top 0.152: R32.2 U6.27
SD_CMD  (via drill 0.25 pad 0.51)
  Top 0.152: U6.28 45.18,27.54 37.02,19.37 37.02,15.3 36.64,14.92 v36.64,14.54
  Bottom 0.152: R27.1 40.76,17.8 40.76,17.39 40.14,16.78 J7.3 40.14,14.62 39.81,14.29 36.89,14.29 v36.64,14.54
SD_D0  (via drill 0.25 pad 0.51)
  Top 0.152: U6.26 41.78,25.15 41.59,24.96 41.46,24.83 36.25,19.62 36.25,15.56 35.62,14.92 v35.62,14.54 | U6.26
  Bottom 0.152: 45.16,17.86 R26.1 44.54,17.27 J7.7 44.54,14.63 43.38,13.46 35.94,13.46 35.62,13.78 v35.62,14.54
SD_D1  (via drill 0.25 pad 0.51)
  Top 0.152: U6.25 40.08,30.14 41.33,28.89 41.33,25.21 35.87,19.75 35.87,15.68 35.11,14.92 v35.11,14.03
  Bottom 0.152: 46.26,17.83 R25.1 45.64,17.22 J7.8 45.64,14.56 44.23,13.14 35.62,13.14 35.11,13.65 v35.11,14.03 35.11,13.78
SD_D2  (via drill 0.25 pad 0.51)
  Top 0.152: 48.58,30.3 U6.30 48.58,29.92 41.59,22.92 41.59,18.35 39.87,16.64 v38.05,16.64
  Bottom 0.152: 38.56,17.85 R29.1 38.54,17.13 v38.05,16.64 37.94,16.53 J7.1
SD_D3  (via drill 0.25 pad 0.51)
  Top 0.152: U6.29 46.92,30.39 46.92,28.77 41.21,23.05 41.21,18.82 v39.66,17.27
  Bottom 0.152: R28.1 39.66,17.84 v39.66,17.27 39.04,16.66 J7.2
SSSS  (via drill 0.25 pad 0.51)
  Top 0.152: v38.03,19.62 37.4,18.99 37.4,14.41 36,13.02 v34.98,13.02
  Bottom 0.152: 47.36,17.79 R24.1 46.74,17.18 J7.9 46.74,14.58 44.99,12.83 35.18,12.83 v34.98,13.02 | Q2.1 37.65,19.68 37.98,19.68 v38.03,19.62
USB_5V  (via drill 0.25 pad 0.51)
  other vias: 25.46,7.68 26.48,6.16 26.86,5.52 25.97,5.52 25.59,6.16 25.08,6.92 25.97,6.92 24.7,9.08 25.97,9.08 25.33,9.08
  pour Bottom (no thermals): 25.97,5.14 26.93,5.14 27.11,5.32 27.11,6.29 26.09,7.3 26.09,8.7 26.22,8.83 26.48,8.83 27.11,9.72 27.11,10.22 26.98,10.35 24.32,10.35 24.19,10.22 24.19,6.92
  pour Top (no thermals): 27.11,3.75 27.11,6.29 26.22,7.18 26.22,8.45 26.73,8.95 26.73,9.72 24.32,9.72 24.19,9.59 24.19,6.92 26.6,4.51 26.6,3.75
USB_M
  Top 0.152: U6.22 34.98,30.29 33.78,29.08 19.68,29.08 18.22,27.62 17.33,27.62 16.43,26.72 J5.16 J5.P$16
USB_P
  Top 0.152: U6.21 33.28,29.61 33.08,29.4 19.49,29.4 18.92,28.83 18.79,28.83 18.35,29.27 18.16,29.27 17.9,29.02 17.9,28.83 18.35,28.38 18.35,28.26 18.03,27.94 17.27,27.94 16.49,28.72 J5.14 J5.P$14
VDD_3V3  (via drill 0.25 pad 0.51)
  Top 0.305: U7.34 19.34,24.79 | U7.14 28.36,20.79 29.27,19.88 v29.27,19.62
  Top 0.508: R53.2 42.1,57.73 v42.16,57.79 | FB2.1 v16.95,18.1 | R1.2 32.44,26.99 v32.83,26.61 | 19.34,24.79 19.3,24.79 C64.2 18.71,24.85 v18.6,24.96 | C63.2 29.65,19.24 v29.27,19.62
  Top 0.813: FB1.1 v26.98,58.36
  PWR 0.305: v29.27,19.62 29.27,19.49 28.95,19.18 27.87,19.18 27.56,19.49
  Bottom 0.254: U5.10 32.66,37.42 v32.51,37.27 | U5.8 34.12,35.4 34.1,35.37
  Bottom 0.305: Q2.2 R29.2 | Q3.2 55.45,51.01 55.05,50.61 54.42,50.61 53.93,50.13 C27.2 | R4.2 57.06,52.28 56.12,53.23 R33.2
  Bottom 0.508: R29.2 R28.2 40.23,18.84 v40.26,18.86 40.28,18.84 R27.2 41.36,18.84 42.07,18.12 C56.1 | R39.2 29.14,42.23 v29.08,42.16 | R38.2 32.55,44.11 v32.51,44.07 | R24.2 R25.2 R26.2 44.87,18.84 43.9,17.87 C57.1 42.5,17.87 | R14.2 v8.5,34.23 | C56.1 42.39,17.91 42.54,17.91 42.5,17.87 | v62.04,39.18 62.04,38.27 R42.2 | R37.2 62.54,36.13 v62.67,36.26 | R35.2 v62.67,34.1 | R8.2 62.67,31.94 62.92,31.69 v62.92,31.05 | R33.2 56.12,54.09 v56.19,54.17 | v52.26,55.44 52.28,55.46 R12.2 R17.2 | R22.2 v10.85,47.82 | v10.85,47.82 | R11.2 v39.29,56.08 v39.3,56.07 | v8.5,37.08 8.57,37.15 R16.2 R15.2 | R13.2 8.44,32.19 v7.43,31.18 | J7.4 41.24,16.61 42.18,17.54 | 42.18,17.54 42.5,17.87 | C56.1 42.18,17.54 | C22.2 32.13,36.89 v32.51,37.27 | 34.1,35.37 C23.2 33.48,34.33 v33.46,34.35
  Bottom 0.61: C27.2 52.66,50.13 v52.64,50.1 | v62.04,39.18 TP2.T
  other vias: 13.65,13.78 13.65,13.14 13.14,13.78 13.14,13.14
  pour Bottom (isolate 0.254, no thermals): 14.54,11.49 13.04,11.49 12.76,11.78 12.76,14.23 12.94,14.41 16.44,14.41 17.59,12.64 17.59,10.54 17.52,10.48 16.7,10.48 16.57,10.6 16.57,11.87 15.93,12.51 15.05,12.51 14.92,12.38 14.92,11.87
  pour PWR (isolate 0.254, rank 6): -2.23,70.42 71.81,70.42 71.81,-3.62 -0.58,-3.62 -0.58,-5.02 -2.23,-5.02
VDD_5V  (via drill 0.25 pad 0.51)
  Top 0.305: U7.2 22.19,17.88 22.03,17.72 | v24.65,17.64 24.69,17.68 U7.7
  Top 0.406: D8.4 33.68,9.69 C17.2 34.23,9.72 v34.35,9.84
  Top 0.508: C74.1 24.95,17.34 v24.65,17.64 | 21.9,16.95 v21.9,16.45 21.52,16.83 | 21.9,16.95 21.9,17.21 | 21.9,17.21 21.9,17.59 22.03,17.72 | 21.52,16.83 16.82,16.83 14.94,18.71 C42.2 13.93,18.71 v13.9,18.73 13,18.73 D10.4 | 21.52,16.83 21.78,16.83 21.9,16.95 | 21.52,16.83 21.9,17.21 | v9.2,30.16 8.97,30.39 C43.2 8.31,32.09 D13.4 | v10.09,43.24 10.09,43.98 C44.2 10.07,44.62 D14.4 | D9.4 23.04,11.12 v22.79,11.37 22.79,11.59 C41.2 | v53.15,12.13 53.12,12.15 C12.2 52.76,10.6 D5.4 | v60,23.43 C11.2 | C11.2 | C11.2 59.22,22.13 D4.4 | v61.27,38.93 61.27,37.78 61.93,37.12 C4.2 61.93,35.64 D3.4 | v57.72,50.48 57.43,50.2 C3.2 57.08,48.45 57.21,48.32 57.21,48.34 D2.4 | v43.75,58.74 45.53,58.74 C1.2 46.67,57.59 D1.4 | D18.4 23.11,56.64 23.81,55.94 C45.2 24.34,56.56 v24.32,56.58 | v32.19,55.31 32.19,58.61 31.81,58.99 C46.2 31.66,59.6 32.4,60.34 D19.4
  Top 0.61: C17.2
  Top 1.016: J6.1 J6.P$1
  PWR 0.254: v40.32,43.5 36.13,43.5 v35.49,44.13
  PWR 0.406: 29.27,13.53 28.63,14.16 | 29.27,13.53 28.51,13.53 28.38,13.4 | 29.27,13.53 29.27,14.41
  PWR 0.508: v13.9,18.73 9.2,23.43 v9.2,30.16 9.2,42.35 v10.09,43.24 | v53.15,12.13 53.15,14.54 60,21.4 v60,23.43 61.91,25.34 61.91,38.29 v61.27,38.93 58.35,41.85 | J6.P$1 55.7,40.72 56.83,41.85 57.72,41.85 | 57.72,41.85 58.35,41.85 | 58.35,41.85 58.35,42.48 | 58.35,42.48 58.35,49.85 v57.72,50.48 55.69,50.48 47.43,58.74 v43.75,58.74 40.83,58.74 36.38,54.29 33.21,54.29 v32.19,55.31 31.68,55.82 25.08,55.82 v24.32,56.58 | 58.35,42.48 57.72,41.85
  PWR 0.61: v30.03,13.02 29.78,13.02 29.27,13.53
  PWR 1.422: v23.43,15.43 23.55,15.3 23.55,14.8 24.44,13.91 28.38,13.91 28.63,14.16 55.19,40.72 J6.P$1
  Bottom 0.254: U5.26 38.71,39.92 40.89,42.1 C51.2 41.21,42.33 C49.1 v40.32,43.5 | U5.21 36.12,44.03 C50.2 35.52,44.16 v35.49,44.13
  Bottom 0.406: U3.2 30.67,14.92 30.02,14.27 U3.5 30.02,13.03 v30.03,13.02 30.03,12.87 C48.2 32.72,12.23 34.35,10.6 v34.35,9.84
  Bottom 0.508: v24.65,17.64 23.96,16.95 TP1.T 23.55,15.56 v23.43,15.43 | U1.1 23.89,11.83 | 23.89,11.83 23.26,11.83 v22.79,11.37 | 23.89,11.83 24.32,12.26
  Bottom 0.61: U4.3 47.05,39.05 46.16,39.94 C14.2 | U4.3 | C14.2 | C14.2 C13.2 44.38,41.97 42.86,43.5 C49.1 | U4.3 52.38,39.05 54.03,40.7 55.56,40.7 J6.P$1
  other vias: 23.81,15.05 23.81,14.03 23.55,14.54
  pour Bottom (no thermals): 17.59,16.52 17.59,15.05 17.71,14.92 22.56,14.92 23.94,13.55 23.94,11.62 24.06,11.49 25.24,11.49 25.33,11.58 25.33,15.81 24.44,16.7 17.76,16.7
VDD_7688
  Top 0.813: FB1.2 27.23,55.89 C60.2 29.49,55.89 C58.1 31.26,56.12 | 31.26,56.12 C59.1 | U6.54 31.58,54.64 31.3,54.93 31.3,56.09 31.26,56.12
VMID
  Bottom 0.152: TP14.T | TP14.T 39.68,39.42
  Bottom 0.254: U5.27 39.68,39.42 40.81,39.42 C54.1
  Bottom 0.406: C54.1 41.08,39.94 41.02,40.01 40.98,40.05 C55.2
WDT_RST_N  (via drill 0.25 pad 0.51)
  Top 0.254: U6.48 41.78,54.1 41.46,54.42 v41.46,55.69 41.44,55.71 R55.2
  Bottom 0.254: K1.1 8.43,49.85 | 8.43,49.85 8.43,49.81 8.26,49.64 | 8.26,49.64 K1.2 | 8.43,49.85 9.5,48.78 R22.1 10.19,48.77 TP12.T 12.51,47.94 22.03,47.94 24.82,50.74 24.82,52.64 | 8.26,49.64 8.65,49.64 8.7,49.59 | 24.82,52.64 24.82,52.9 | 24.82,52.9 24.82,53.15 | 24.82,53.15 24.82,55.18 25.33,55.69 29.02,55.69 32.48,59.16 BUTTON1.3 | 25.08,52.9 39.18,52.9 41.46,55.18 v41.46,55.69 | 25.08,52.9 24.82,52.9 | 25.08,52.9 24.82,53.15 | 25.08,52.9 24.82,52.64
WLED_N  (via drill 0.25 pad 0.51)
  Top 0.152: U6.45 46.88,56.03 49.97,59.12 v51.75,59.12
  Bottom 0.152: v51.75,59.12 51.75,59.32 D12.2

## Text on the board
Top: 1
GND: 2
PWR: 3
Bottom: 4
bNames: Respeaker Core | v1.0 10/13/2016
tTest: 5V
